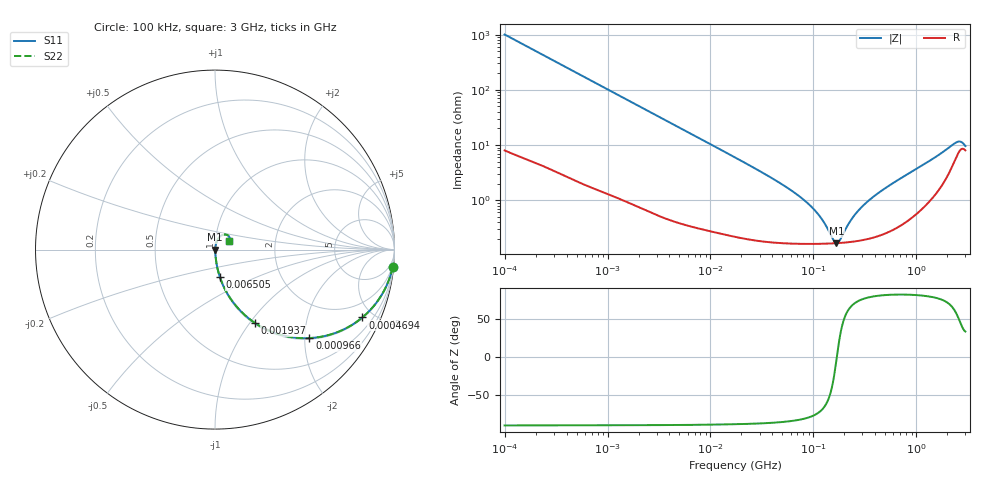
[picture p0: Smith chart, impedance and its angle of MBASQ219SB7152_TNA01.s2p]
! MBASQ219SB7152_TNA01  S-PARAMETER MODEL  ( Standard Model )
! Model Generated by TAIYO YUDEN Corporation (http://www.ty-top.com)
! Version 1.0
! TAIYO YUDEN Control No. 220601
! Copyright(c) 2013 TAIYO YUDEN CO.,LTD. All Rights Reserved.
! Product Description (link to TY-COMPAS)
! https://ds.yuden.co.jp/TYCOMPAS/or/detail?pn=MBASQ219SB7152KTNA01&u=M
! Products Name : Multilayer Ceramic Capacitors
! Characteristics :
!  Capacitance : 1500 [pF] , Rated Voltage : 250 [V] , TCC : X7R
!  Case Size : 2.0 x 1.25 / 0.079 x 0.049 [mm/inch] , Thickness : 0.85 / 0.033 [mm/inch]
!  (Conditions: Temperature = 25 [degC] , DC Bias Voltage = 0 [V])
! External Node Assignments :
!  1  o---| |---o  2
! GND o---------o GND
! Frequency Range : 100kHz  -  3GHz  [ 401 STEP ]
# MHZ S RI R 50
! Freq[MHz].  S11 Real  S11 Imag  S21 Real  S21 Imag  S12 Real  S12 Imag  S22 Real  S22 Imag
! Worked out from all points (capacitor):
!   401 points, 100 kHz to 3 GHz, reference 50 ohm
!   read as one part in series: C = 1.58 nF near 105.3 kHz
!   lowest |Z| = 167 mohm at 167.3 MHz (marker M1)
!   series resonance near 169 MHz, so ESL is about 560 pH
!   S11 on the Smith chart (normalised r, x): 100 kHz: 1, -20; 469.4 kHz: 1.05, -4.32; 966 kHz: 1.03, -2.11; 1.937 MHz: 1.02, -1.06; 6.505 MHz: 1.01, -0.32; 3 GHz: 1.16, +0.11
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0.1  0.9894 -0.0983  0.0106 0.0983  0.0106 0.0983  0.9894 -0.0983
0.246461  0.9418 -0.2292  0.0582 0.2292  0.0582 0.2292  0.9418 -0.2292
0.469427  0.821 -0.378  0.179 0.378  0.179 0.378  0.821 -0.378
0.562235  0.7629 -0.4198  0.2371 0.4198  0.2371 0.4198  0.7629 -0.4198
0.965977  0.5265 -0.493  0.4735 0.493  0.4735 0.493  0.5265 -0.493
1.937191  0.2221 -0.4085  0.7779 0.4085  0.7779 0.4085  0.2221 -0.4085
3.161081  0.0995 -0.2915  0.9005 0.2915  0.9005 0.2915  0.0995 -0.2915
6.504802  0.0276 -0.1538  0.9724 0.1538  0.9724 0.1538  0.0276 -0.1538
17.7727  0.00548 -0.0576  0.9945 0.0576  0.9945 0.0576  0.00548 -0.0576
53.83243  0.00195 -0.0174  0.998 0.0174  0.998 0.0174  0.00195 -0.0174
97.38194  0.00166 -0.00718  0.9983 0.00718  0.9983 0.00718  0.00166 -0.00718
119.6798  0.00164 -0.00436  0.9984 0.00436  0.9984 0.00436  0.00164 -0.00436
154.8634  0.00165 -0.00108  0.9983 0.00108  0.9983 0.00108  0.00165 -0.00108
167.3121  0.00166 -0.000124  0.9983 0.000124  0.9983 0.000124  0.00166 -0.000124
180.7614  0.00168 0.000835  0.9983 -0.000835  0.9983 -0.000835  0.00168 0.000835
227.9507  0.00176 0.00377  0.9982 -0.00377  0.9982 -0.00377  0.00176 0.00377
280.1453  0.00189 0.00654  0.9981 -0.00654  0.9981 -0.00654  0.00189 0.00654
371.9668  0.00218 0.0108  0.9978 -0.0108  0.9978 -0.0108  0.00218 0.0108
547.5153  0.00301 0.0182  0.997 -0.0182  0.997 -0.0182  0.00301 0.0182
2378.954  0.0584 0.0841  0.9416 -0.0841  0.9416 -0.0841  0.0584 0.0841
2637.286  0.0784 0.073  0.9216 -0.073  0.9216 -0.073  0.0784 0.073
3000  0.0762 0.0453  0.9238 -0.0453  0.9238 -0.0453  0.0762 0.0453
